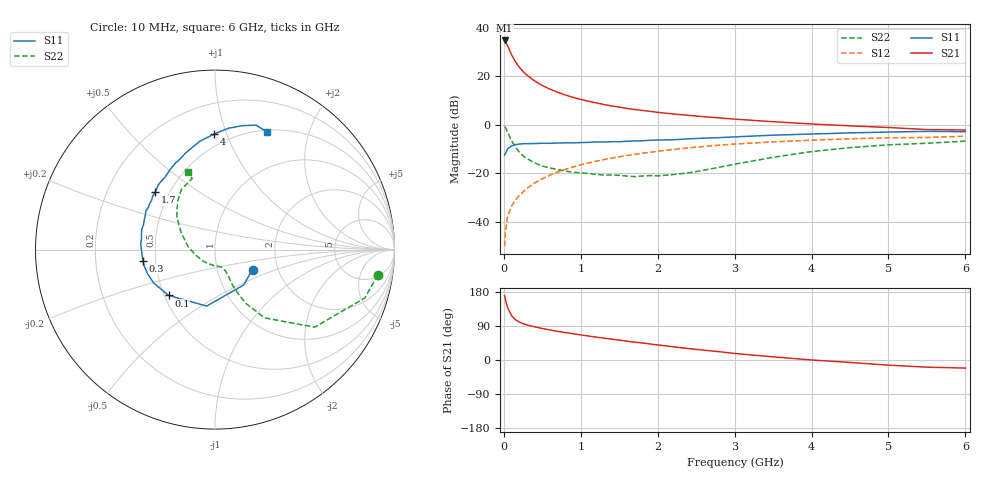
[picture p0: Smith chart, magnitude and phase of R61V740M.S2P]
! SIEMENS Small Signal Semiconductors
! BFR193
! Si NPN RF Bipolar Junction Transistor in SOT23
! VCE = 1.75 V  IC = 40 mA
! Common Emitter S-Parameters:  May  1996
# GHz  S  MA  R  50
!  f  S11  S21  S12  S22
! GHz  MAG  ANG  MAG  ANG  MAG  ANG  MAG  ANG
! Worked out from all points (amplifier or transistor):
!   36 points, 10 MHz to 6 GHz, reference 50 ohm
!   highest |S21| = 34.8 dB at 10 MHz (marker M1)
!   |S21| within 3 dB of that: start of sweep to 60.17 MHz
!   unconditionally stable (mu >= 1): 382.2 MHz to 1.88 GHz
!   at 250 MHz: K = 0.95, MSG = 24.9 dB, |S12| = -27.7 dB
!   at 1.4 GHz: K = 1.03, MAG = 9.8 dB, |S12| = -13.8 dB
!   at 6 GHz: K = 0.96, MSG = 1.3 dB, |S12| = -4.7 dB
!   S11 on the Smith chart (normalised r, x): 10 MHz: 1.48, -0.35; 100 MHz: 0.53, -0.31; 300 MHz: 0.42, -0.06; 1.7 GHz: 0.42, +0.34; 4 GHz: 0.41, +0.90; 6 GHz: 0.52, +1.40
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0.01  0.237 -28.0  55.21 169.7  0.0031 85.6  0.9175 -8.8
0.02  0.2538 -51.0  53.09 159.9  0.0061 77.8  0.8773 -17.9
0.05  0.3181 -98.4  42.55 137.5  0.0131 70.9  0.7036 -37.9
0.1  0.3634 -135.3  28.02 117.2  0.0209 67.3  0.4703 -54.0
0.15  0.3897 -151.7  20.15 106.5  0.0279 68.2  0.3449 -60.2
0.2  0.399 -160.6  15.6 100.2  0.0343 70.7  0.2749 -62.4
0.25  0.405 -167.0  12.59 95.9  0.0412 71.7  0.2281 -63.6
0.3  0.4069 -171.3  10.61 92.5  0.0486 72.5  0.1999 -63.6
0.4  0.4087 -178.6  8.06 87.6  0.0627 73.3  0.1638 -63.3
0.5  0.4148 176.2  6.476 83.2  0.0765 73.3  0.1398 -63.6
0.6  0.4141 171.4  5.432 79.3  0.0912 72.8  0.1276 -64.4
0.7  0.4198 167.6  4.686 75.6  0.1056 71.9  0.1187 -65.7
0.8  0.4232 164.2  4.12 72.4  0.1199 70.7  0.1105 -67.5
1.1  0.4329 153.8  3.067 63.3  0.1628 67.1  0.0986 -76.2
1.4  0.4458 144.5  2.449 55.1  0.204 62.8  0.0914 -87.8
1.7  0.4621 136.2  2.07 47.0  0.2441 58.3  0.0848 -104.6
2.2  0.4896 124.6  1.672 35.0  0.3086 50.6  0.0934 -138.5
3.5  0.6097 98.0  1.156 8.3  0.4429 29.6  0.2127 152.9
4  0.6429 90.5  1.038 0.1  0.4805 22.5  0.279 139.7
4.5  0.6795 83.9  0.95 -6.5  0.5136 15.4  0.3371 128.5
5.5  0.7302 71.8  0.796 -18.9  0.5465 1.6  0.4151 107.8
6  0.718 66.4  0.779 -21.3  0.5803 -2.5  0.459 109.4
